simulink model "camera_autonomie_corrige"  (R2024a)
settings: Solver=ode14x  StartTime=0.0  StopTime=86400  FixedStep=60  RelTol=1e-3  EnableMultiTasking=on
libraries: nesl_utility x8, fl_lib x7, SignalEditorBlockLib x2, ee_lib x2, batteryecm_lib x1

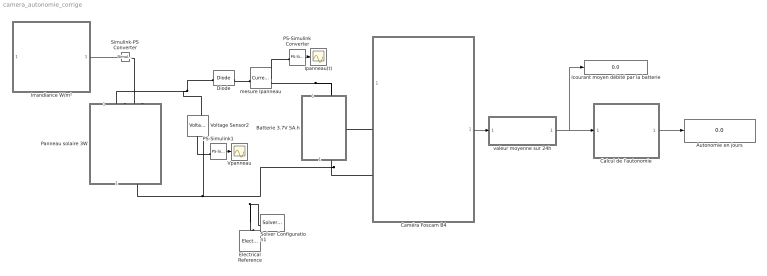
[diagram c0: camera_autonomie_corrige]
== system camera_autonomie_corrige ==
  Autonomie en jours : Display
  Batterie 3.7V 5A.h : Subsystem  mask{tension=3.7, capacite=5, resistance=0.02}
      mask prompts: tension "Tension nominale (V)"; capacite "Capacité nominale (A.h)"; resistance "Résistance interne (Ohm)"
  Calcul de l'autonomie : Subsystem
  Caméra Foscam B4 : Subsystem
  Diode : ee_lib/Semiconductors & Converters/Diode  ModelType=ee.enum.diode.modelType.pwl  TableType=ee.enum.diode.tableType.IfMat  IfMat=[.07, .12, .19, 1.75, 4.24, 7.32, 11.2; .16, .3, .72, 2.14, 5.02, 8.35, 13.12] A  VfMat=[.9, 1.15, 1.25, 1.5, 1.75, 2.17, 2.6, 2.85; .58, .68, .75, 1.1, 1.38, 1.77, 2.27, 2.7] V  TjVec=[25, 125] degC  VfVec=[.5, .7, .9, 1.3, 1.7, 2.1, 2.5] V  IfVec=[.1, .2, .5, 1, 2, 4, 7, 10] A  IrMat=[1e-06, 2e-06, 5e-06, 1e-05, 2.5e-05, 5e-05, .0001; 2e-06, 5e-06, 1e-05, 4e-05, 8e-05, .0002, .0005] A  VrMat=[10, 100, 200, 250, 300, 325, 350; 10, 70, 160, 220, 270, 300, 320] V  VrVec=[10, 20, 40, 50, 70, 80, 100] V  IrVec=[1e-06, 2e-06, 5e-06, 1e-05, 2e-05, 5e-05, .0001] A  Vf=0.15 V  Ron=0.03 Ohm  Goff=1e-8 S  prmExp=ee.enum.diode.expParam.useTwo  I12=[.0137, .545] A  V12=[.6, .7] V  RS=0 Ohm  Tmeas=25 degC  IS=1e-12 A  ec=1  I1=0.0137 A  V1=0.6 V  N_series=1  N_parallel=1  ZenerEnable=false  Rz=0.3 Ohm  BV=inf V  C_param=ee.enum.diode.capParam.fixed  CJ=5 pF  CJ0=5 pF  Vvec=[.1, 10, 100] V  Cvec=[3.5, 1, .4] pF  VJ=1 V  Mgrad=0.5  FC=0.5  Q_param=ee.enum.diode.recoveryParam.off  iRM=-7.15 A  iF=4 A  didt=-750 A/us  trr_factor=3  trr=115 ns  Qrr=150 nA*s  Vr=-600 V  Ls=150 nH  Erec=0.03 J  TT=50 ns  tau=100 ns  T_param=ee.enum.diode.temperatureParam.off  Tdevice=25 degC  I1_T2=0.245 A  V1_T2=0.5 V  IS_T2=1.25e-7 A  Tmeas2=125 degC  XTI_param=ee.enum.diode.xtiParam.pn  XTI=3  EG_param=ee.enum.diode.egapParam.material_si  EG=1.11 eV  dBVdT=0 V/K  enable_faults=ee.enum.enable.no  fault_action=simscape.enum.assert.action.none  fault_types=ee.enum.diode.faults.open  tau_fault=1e-3 s  IfMat_faulted=[.07, .12, .19, 1.75, 4.24, 7.32, 11.2; .16, .3, .72, 2.14, 4.02, 6.35, 9.12] A  VfMat_faulted=[.9, 1.15, 1.25, 1.5, 1.75, 2.17, 2.6, 2.85; .58, .68, .75, 1.1, 1.38, 1.77, 2.27, 2.7] V  VfVec_faulted=[.5, .7, .9, 1.3, 1.7, 2.1, 2.5] V  IfVec_faulted=[.1, .2, .5, 1, 2, 4, 7, 10] A  IrMat_faulted=[1e-06, 2e-06, 5e-06, 1e-05, 2.5e-05, 5e-05, .0001; 2e-06, 5e-06, 1e-05, 4e-05, 8e-05, .0002, .0005] A  VrMat_faulted=[1, 10, 20, 25, 30, 32.5, 35; 1, 5, 10, 20, 25, 30, 32] V  VrVec_faulted=[1, 2, 4, 5, 7, 8, 10] V  IrVec_faulted=[1e-06, 2e-06, 5e-06, 1e-05, 2e-05, 5e-05, .0001] A  Ropen_faulted=1000 Ohm  Gshort_faulted=1000 1/Ohm  Vf_faulted=0.6 V  Ron_faulted=0.3 Ohm  Goff_faulted=1e-8 S  I12_faulted=[.0137, .545] A  V12_faulted=[.6, .7] V  IS_faulted=1e-12 A  ec_faulted=1  I1_faulted=0.0137 A  V1_faulted=0.6 V  RS_faulted=0 Ohm  Rz_faulted=0.3 Ohm  BV_faulted=inf V  Cscale_faulted=100  fault_trigger=ee.enum.faults.faultTrigger.temporal  t_fault=inf s  max_permissible_voltage=inf V  n_fail_on_voltage=1  max_permissible_current=inf A  t_fail_on_current=1 s  max_permissible_dVdt=inf V/s  enable_fault_input=simscape.enum.onoff.off  i_specify=off  i_priority=None  i=0 A  i_nominal_specify=off  i_nominal_value=1  i_nominal_unit=A  v_specify=off  v_priority=None  v=0 V  v_nominal_specify=off  v_nominal_value=1  v_nominal_unit=V  v_capacitor_specify=off  v_capacitor_priority=None  v_capacitor=0 V  v_capacitor_nominal_specify=off  v_capacitor_nominal_value=1  v_capacitor_nominal_unit=V  Qj_specify=off  Qj_priority=High  Qj=0 C  Qj_nominal_specify=off  Qj_nominal_value=1  Qj_nominal_unit=C  faulted_specify=off  faulted_priority=None  faulted=0  faulted_nominal_specify=off  faulted_nominal_value=1  faulted_nominal_unit=1  i_diode_specify=off  i_diode_priority=None  i_diode=0 A  i_diode_nominal_specify=off  i_diode_nominal_value=1  i_diode_nominal_unit=A  v_diode_specify=off  v_diode_priority=None  v_diode=0 V  v_diode_nominal_specify=off  v_diode_nominal_value=1  v_diode_nominal_unit=V  i_capacitor_specify=off  i_capacitor_priority=None  i_capacitor=0 A  i_capacitor_nominal_specify=off  i_capacitor_nominal_value=1  i_capacitor_nominal_unit=A  power_dissipated_specify=off  power_dissipated_priority=None  power_dissipated=0 W  power_dissipated_nominal_specify=off  power_dissipated_nominal_value=1  power_dissipated_nominal_unit=W  fidelity_level=ee.enum.diode.fidelity.includeChargeDyn  rec_loss_model=ee.enum.diode.reverseRecoveryModel.fixed  ErecVal=0 J  scaleWithIandV=true  ErecMat=zeros(2, 3) J  TjrecVec=[298.15, 398.15] K  IfrecVec=[.1, 1, 10] A  IrecVal=10 A  VrecVal=10 V  tFilter=1 / 1000 / 100 s  max_permissible_temperature=inf K  t_fail_on_temperature=1 s  thermal_network_parameterization=ee.enum.thermalNetworkTopology.junctionCase  Rth=[0, 10] K/W  Rth_Cauer=[1, 3, 10] K/W  Rth_Foster=[4, 6] K/W  thermal_mass_parameterization=ee.enum.thermalNetwork.timeconstant  thermal_mass=[0, 1] J/K  thermal_mass_Cauer=[.1, .3, 1] J/K  thermal_mass_Foster=[1.5, 3] J/K  thermal_time_constant=[0, 10] s  thermal_time_constant_Cauer=[1, 3, 10] s  thermal_time_constant_Foster=[6, 18] s  thermal_mass_initial_temperatures=[25, 25] degC  thermal_mass_initial_temperatures_Cauer=[25, 25, 25] degC  junction_thermal_mass=0.01 J/K  Tvec_initial_Foster=[25, 25, 25, 25] degC  no_thermal_network=0  junction_temperature_specify=off  junction_temperature_priority=None  junction_temperature=25 degC  junction_temperature_nominal_specify=off  junction_temperature_nominal_value=1  junction_temperature_nominal_unit=degC
  Electrical Reference : fl_lib/Electrical/Electrical Elements/Electrical Reference
  Icourant moyen débité par la batterie : Display
  Ipanneau(t) : Scope
  Irrandiance W/m² : Subsystem
  PS-Simulink Converter : nesl_utility/PS-Simulink Converter  PhysicalDomain=network_engine_domain  SubClassName=ps_output  LeftPortType=input  RightPortType=output  PseudoPeriodic=off  Frequencies=[]  VectorFormat=1-D array  Unit=A  AffineConversion=off
  PS-Simulink1 : nesl_utility/PS-Simulink Converter  PhysicalDomain=network_engine_domain  SubClassName=ps_output  LeftPortType=input  RightPortType=output  PseudoPeriodic=off  Frequencies=[]  VectorFormat=1-D array  Unit=V  AffineConversion=on
  Panneau solaire 3W : Subsystem  mask{Isc=0.45, Voc=7, facteur=1.5}
      mask prompts: Isc "Courant de court-circuit Isc(A)"; Voc "Tension en circuit ouvert Voc(V)"; facteur "Facteur de qualité"
  Simulink-PS Converter : nesl_utility/Simulink-PS Converter  PhysicalDomain=network_engine_domain  SubClassName=ps_input  LeftPortType=input  RightPortType=output  PseudoPeriodic=off  Frequencies=[]  NoiseDistribution=none  NoiseParameters=[]  Unit=1  AffineConversion=off  FilteringAndDerivatives=provide  SimscapeFilterOrder=1  InputFilterTimeConstant=0.001  UdotUserProvided=0
  Solver Configuration1 : nesl_utility/Solver Configuration  PhysicalDomain=network_engine_domain  SubClassName=solver  LeftPortType=input  RightPortType=generic  Tones=[]  Harmonics=[]  SimulateNoise=off  Profile=off  UseLocalSampling=off  EnableSwitchedLinearOptims=on  FrequencyDomain=off  UseCCode=off  RelTol=0.001  AbsTol=0.001  MinStep=1e-09  ToWorkspace=off  RevertToSquareIcSolve=off  NumHomotopyIterations=100  PhasorMode=off  PhasorModeNumHarmonics=1  ConsistencySolver=NEWTON_XTOL_AFTER_FTOL  IndexReductionMethod=DerivativeReplacement  DoDC=off  ResidualTolerance=1e-09  ConsistencyTolSource=GLOBAL  ConsistencyAbsTol=0.001  ConsistencyRelTol=0.001  ConsistencyTolFactor=0.001  UseLocalSolver=off  LocalSolverChoice=NE_BACKWARD_EULER_ADVANCER  ResolveIndetEquations=on  FunctionEvalNumThread=1  LocalSolverSampleTime=0.001  DoFixedCost=off  MaxNonlinIter=3  MaxModeIter=2  ComputeImpulses=off  ImpulseIterations=2  LinearAlgebra=auto  LinearAlgebraNumThread=0  EquationFormulation=NE_TIME_EF  DelaysMemoryBudget=1024  AutomaticFiltering=on  FilteringTimeConstant=0.001  PartitionStorageMethod=AS_NEEDED  PartitionMemoryBudget=1024  PartitionMethod=ROBUST  MultibodyUseLocalSolver=off  MultibodyLocalSolverChoice=ODE1  MultibodyLocalSolverSampleTime=0.001
  Voltage Sensor2 : fl_lib/Electrical/Electrical Sensors/Voltage Sensor
  Vpanneau : Scope
  mesure Ipanneau : fl_lib/Electrical/Electrical Sensors/Current Sensor
  valeur moyenne sur 24h : Subsystem
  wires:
  PS-Simulink1/1 -> Vpanneau/1
  PS-Simulink Converter/1 -> Ipanneau(t)/1
  valeur moyenne sur 24h/1(Out1) -> Icourant moyen débité par la batterie/1, Calcul de l'autonomie/1(In1)
  Caméra Foscam B4/1(Courant (A)) -> valeur moyenne sur 24h/1(In1)
  Irrandiance W/m²/1(Irradiance W/m²) -> Simulink-PS Converter/1
  Calcul de l'autonomie/1(Out1) -> Autonomie en jours/1
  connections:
  mesure Ipanneau/RConn1 -- PS-Simulink Converter/LConn1
  Panneau solaire 3W/RConn1 -- Solver Configuration1/RConn1 -- Electrical Reference/LConn1 -- Batterie 3.7V 5A.h/RConn1 -- Caméra Foscam B4/LConn2 -- Voltage Sensor2/RConn2
  mesure Ipanneau/RConn2 -- Caméra Foscam B4/LConn1 -- Batterie 3.7V 5A.h/LConn1
  Diode/RConn1 -- mesure Ipanneau/LConn1
  Diode/LConn1 -- Panneau solaire 3W/LConn1 -- Voltage Sensor2/LConn1
  Voltage Sensor2/RConn1 -- PS-Simulink1/LConn1
  Simulink-PS Converter/RConn1 -- Panneau solaire 3W/LConn2

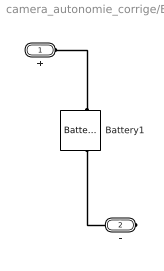
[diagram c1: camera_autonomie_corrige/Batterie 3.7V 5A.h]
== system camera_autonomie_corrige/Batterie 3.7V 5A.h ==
  Battery1 : batteryecm_lib/Battery  Vnom=tension V  prm_dir=simscape.enum.battery.prm_dir.disabled  R1_dis=2 Ohm  R1_ch=2 Ohm  R1=resistance Ohm  prm_AH=simscape.enum.battery.prm_AH.finite  AH=capacite A*hr  V1=3 V  AH1=0.8 A*hr  prm_R2=simscape.enum.battery.prm_R2.disabled  R2=2000 Ohm  Tmeas=298.15 K  charge_measurement_port=simscape.enum.battery.enable.no  prm_dyn=simscape.enum.battery.prm_dyn.off  Rp1=0.005 Ohm  tau1=30 s  Rp2=0.005 Ohm  tau2=30 s  Rp3=0.005 Ohm  tau3=30 s  Rp4=0.005 Ohm  tau4=30 s  Rp5=0.005 Ohm  tau5=30 s  prm_fade=simscape.enum.battery.prm_fade.disabled  N_fade=100  AH_fade=45 A*hr  R1_fade=2.02 Ohm  R1_ch_fade=2.02 Ohm  V1_fade=10.35 V  prm_age=simscape.enum.battery.prm_age.disabled  prm_age_OCV=simscape.enum.battery.prm_age_OCV.OCV  OCV_age=0.9  SOC_age=60  Tmeas_age=298.15 K  delta_time_age_vec=[0] d  temperature_age_vec=[273] K  OCV_scaling_age=2.2134e6  OCV_offset_age=1.632e6  temp_exp_age=0.515833569 V  t_exp_age=0.75  Vnom_T2=12 V  R1_T2=2.2 Ohm  R1_T2_dis=2.2 Ohm  R1_T2_ch=2.2 Ohm  V1_T2=11.4 V  R2_T2=2200 Ohm  Rp1_T2=0.005 Ohm  tau1_T2=30 s  Rp2_T2=0.005 Ohm  tau2_T2=30 s  Rp3_T2=0.005 Ohm  tau3_T2=30 s  Rp4_T2=0.005 Ohm  tau4_T2=30 s  Rp5_T2=0.005 Ohm  tau5_T2=30 s  Tmeas2=273.15 K  thermal_port=simscape.enum.thermaleffects.omit  thermal_mass=30000 J/K  i_specify=off  i_priority=None  i=0 A  i_nominal_specify=off  i_nominal_value=1  i_nominal_unit=A  v_specify=off  v_priority=None  v=0 V  v_nominal_specify=off  v_nominal_value=1  v_nominal_unit=V  charge_specify=off  charge_priority=High  charge=50 A*hr  charge_nominal_specify=off  charge_nominal_value=1  charge_nominal_unit=A*hr  num_cycles_specify=off  num_cycles_priority=High  num_cycles=0  num_cycles_nominal_specify=off  num_cycles_nominal_value=1  num_cycles_nominal_unit=1  temperature_specify=off  temperature_priority=High  temperature=298.15 K  temperature_nominal_specify=off  temperature_nominal_value=1  temperature_nominal_unit=K
  + : PMIOPort  Side=Left
  - : PMIOPort  Port=2  Side=Right
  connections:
  Battery1/RConn1 -- -/RConn1
  Battery1/LConn1 -- +/RConn1

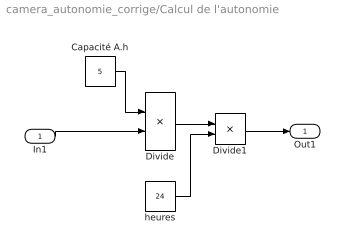
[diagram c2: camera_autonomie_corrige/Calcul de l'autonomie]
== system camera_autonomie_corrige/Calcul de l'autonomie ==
  In1 : Inport
  Capacité A.h : Constant  Value=5
  Divide : Product  Inputs=*/
  Divide1 : Product  Inputs=*/
  heures : Constant  Value=24
  Out1 : Outport
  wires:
  In1/1 -> Divide/2
  Capacité A.h/1 -> Divide/1
  Divide/1 -> Divide1/1
  Divide1/1 -> Out1/1
  heures/1 -> Divide1/2

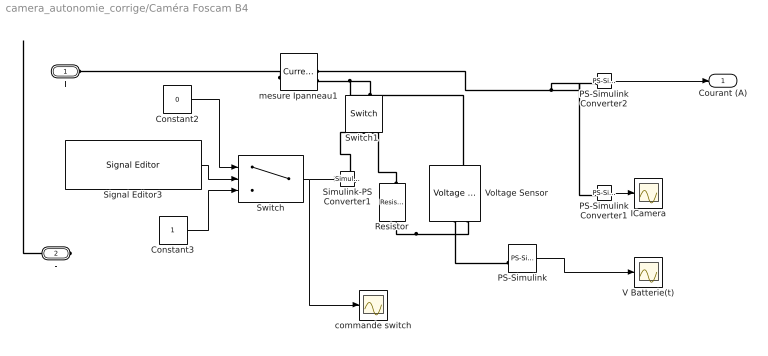
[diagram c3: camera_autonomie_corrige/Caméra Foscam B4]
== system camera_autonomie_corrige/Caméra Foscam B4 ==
  Constant2 : Constant  Value=0
  Constant3 : Constant
  ICamera : Scope
  PS-Simulink : nesl_utility/PS-Simulink Converter  PhysicalDomain=network_engine_domain  SubClassName=ps_output  LeftPortType=input  RightPortType=output  PseudoPeriodic=off  Frequencies=[]  VectorFormat=1-D array  Unit=V  AffineConversion=on
  PS-Simulink Converter1 : nesl_utility/PS-Simulink Converter  PhysicalDomain=network_engine_domain  SubClassName=ps_output  LeftPortType=input  RightPortType=output  PseudoPeriodic=off  Frequencies=[]  VectorFormat=1-D array  Unit=inherit  AffineConversion=off
  PS-Simulink Converter2 : nesl_utility/PS-Simulink Converter  PhysicalDomain=network_engine_domain  SubClassName=ps_output  LeftPortType=input  RightPortType=output  PseudoPeriodic=off  Frequencies=[]  VectorFormat=1-D array  Unit=A  AffineConversion=off
  Resistor : fl_lib/Electrical/Electrical Elements/Resistor  R=50 Ohm  i_specify=off  i_priority=None  i=0 A  i_nominal_specify=off  i_nominal_value=1  i_nominal_unit=A  v_specify=off  v_priority=None  v=0 V  v_nominal_specify=off  v_nominal_value=1  v_nominal_unit=V
  Signal Editor3 : SignalEditorBlockLib/Signal Editor  FileName=courant_consomme.mat  ActiveScenario=Scenario  ActiveSignal=consommation_courant  IsBus=off  OutputBusObjectStr=Bus: BusObject  SampleTime=0  Interpolate=off  ZeroCross=off  OutputAfterFinalValue=Setting to zero  Unit=inherit  PreserveSignalName=on  ApplySigPropsToAllScenarios=on  ApplySigPropsToAllSignals=off
  Simulink-PS Converter1 : nesl_utility/Simulink-PS Converter  PhysicalDomain=network_engine_domain  SubClassName=ps_input  LeftPortType=input  RightPortType=output  PseudoPeriodic=off  Frequencies=[]  NoiseDistribution=none  NoiseParameters=[]  Unit=1  AffineConversion=off  FilteringAndDerivatives=provide  SimscapeFilterOrder=1  InputFilterTimeConstant=0.001  UdotUserProvided=0
  Switch : Switch  Criteria=u2 > Threshold  Threshold=-0.1
  Switch1 : fl_lib/Electrical/Electrical Elements/Switch  R_closed=0.01 Ohm  G_open=1e-8 1/Ohm  Threshold=0.5  i_specify=off  i_priority=None  i=0 A  i_nominal_specify=off  i_nominal_value=1  i_nominal_unit=A  v_specify=off  v_priority=None  v=0 V  v_nominal_specify=off  v_nominal_value=1  v_nominal_unit=V
  V Batterie(t) : Scope
  Voltage Sensor : fl_lib/Electrical/Electrical Sensors/Voltage Sensor
  commande switch : Scope
  mesure Ipanneau1 : fl_lib/Electrical/Electrical Sensors/Current Sensor
  + : PMIOPort  Side=Left
  - : PMIOPort  Port=2  Side=Left
  Courant (A) : Outport
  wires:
  PS-Simulink/1 -> V Batterie(t)/1
  Switch/1 -> commande switch/1, Simulink-PS Converter1/1
  Constant2/1 -> Switch/1
  PS-Simulink Converter1/1 -> ICamera/1
  Constant3/1 -> Switch/3
  Signal Editor3/1 -> Switch/2
  PS-Simulink Converter2/1 -> Courant (A)/1
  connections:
  Voltage Sensor/RConn1 -- PS-Simulink/LConn1
  mesure Ipanneau1/RConn2 -- Voltage Sensor/LConn1 -- Switch1/LConn1
  Voltage Sensor/RConn2 -- -/RConn1 -- Resistor/RConn1
  Resistor/LConn1 -- Switch1/RConn2
  mesure Ipanneau1/RConn1 -- PS-Simulink Converter1/LConn1 -- PS-Simulink Converter2/LConn1
  Simulink-PS Converter1/RConn1 -- Switch1/RConn1
  mesure Ipanneau1/LConn1 -- +/RConn1

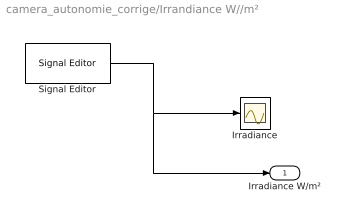
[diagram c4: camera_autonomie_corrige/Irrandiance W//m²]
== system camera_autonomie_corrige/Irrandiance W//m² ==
  Irradiance : Scope
  Signal Editor : SignalEditorBlockLib/Signal Editor  FileName=irradiance_V2.mat  ActiveScenario=ScenarioIrradiance  ActiveSignal=Signal 1  IsBus=off  OutputBusObjectStr=Bus: BusObject  SampleTime=0  Interpolate=off  ZeroCross=off  OutputAfterFinalValue=Setting to zero  Unit=inherit  PreserveSignalName=on  ApplySigPropsToAllScenarios=on  ApplySigPropsToAllSignals=off
  Irradiance W/m² : Outport
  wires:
  Signal Editor/1 -> Irradiance W/m²/1, Irradiance/1

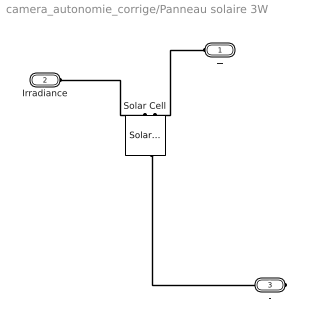
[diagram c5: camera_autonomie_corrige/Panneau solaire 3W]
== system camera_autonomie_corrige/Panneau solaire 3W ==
  Solar Cell : ee_lib/Sources/Solar Cell  prm=1  Isc=Isc A  Voc=Voc V  Is=1e-6 A  Is2=0 A  Iph=7.34 A  Ir0=800 W/m^2  ec=facteur  N2=2  Rs=1 Ohm  Rp=inf Ohm  N_series=1  N_parallel=1  TIPH1=0 1/K  EG=1.11 eV  TXIS1=3  TXIS2=3  TRS1=0  TRP1=0  Tmeas=25 degC  TFIXED=25 degC  thermal_mass=100 J/K  initial_temperature=25 degC
  + : PMIOPort  Side=Left
  Irradiance : PMIOPort  Port=2  Side=Left
  - : PMIOPort  Port=3  Side=Right
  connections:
  Irradiance/RConn1 -- Solar Cell/LConn1
  +/RConn1 -- Solar Cell/LConn2
  Solar Cell/RConn1 -- -/RConn1

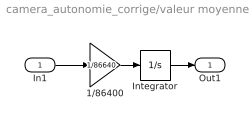
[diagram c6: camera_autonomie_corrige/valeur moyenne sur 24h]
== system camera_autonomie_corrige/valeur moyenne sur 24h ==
  In1 : Inport
  1/86400 : Gain  Gain=1/86640
  Integrator : Integrator
  Out1 : Outport
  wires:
  1/86400/1 -> Integrator/1
  In1/1 -> 1/86400/1
  Integrator/1 -> Out1/1
